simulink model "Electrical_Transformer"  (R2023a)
settings: Solver=VariableStepAuto  StartTime=0.0  StopTime=10.0  RelTol=1e-3
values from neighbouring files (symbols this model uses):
  R = 1    [Electrical_Transformer_EQN.m]    (also in Electrical_Transformer_SLX_m.m; Mechanical_Transmission_EQN.m; Mechanical_Transmission_SLX_m.m; Mechanical_system_EQN.m)
undefined symbols (not defined in the file or in its folder): eTe
libraries: fl_lib x9

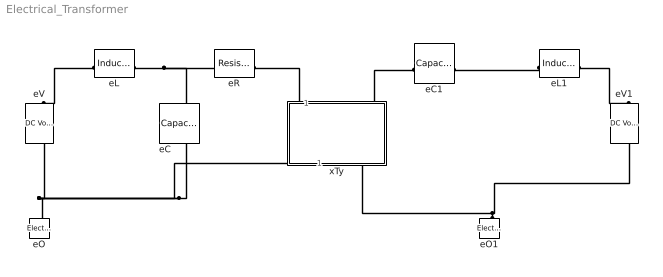
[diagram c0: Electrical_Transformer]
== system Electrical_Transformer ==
  eC : fl_lib/Electrical/Electrical Elements/Capacitor  c=1e-6 F  r=1e-6 Ohm  g=0 1/Ohm  i_specify=off  i_priority=None  i=0 A  i_nominal_specify=off  i_nominal_unit=A  i_nominal_value=1  v_specify=off  v_priority=None  v=0 V  v_nominal_specify=off  v_nominal_unit=V  v_nominal_value=1  vc_specify=off  vc_priority=High  vc=0 V  vc_nominal_specify=off  vc_nominal_unit=V  vc_nominal_value=1
  eC1 : fl_lib/Electrical/Electrical Elements/Capacitor  c=1e-6 F  r=1e-6 Ohm  g=0 1/Ohm  i_specify=off  i_priority=None  i=0 A  i_nominal_specify=off  i_nominal_unit=A  i_nominal_value=1  v_specify=off  v_priority=None  v=0 V  v_nominal_specify=off  v_nominal_unit=V  v_nominal_value=1  vc_specify=off  vc_priority=High  vc=0 V  vc_nominal_specify=off  vc_nominal_unit=V  vc_nominal_value=1
  eL : fl_lib/Electrical/Electrical Elements/Inductor  l=1e-6 H  r=0 Ohm  g=1e-9 1/Ohm  i_specify=off  i_priority=None  i=0 A  i_nominal_specify=off  i_nominal_unit=A  i_nominal_value=1  v_specify=off  v_priority=None  v=0 V  v_nominal_specify=off  v_nominal_unit=V  v_nominal_value=1  i_L_specify=off  i_L_priority=High  i_L=0 A  i_L_nominal_specify=off  i_L_nominal_unit=A  i_L_nominal_value=1
  eL1 : fl_lib/Electrical/Electrical Elements/Inductor  l=1e-6 H  r=0 Ohm  g=1e-9 1/Ohm  i_specify=off  i_priority=None  i=0 A  i_nominal_specify=off  i_nominal_unit=A  i_nominal_value=1  v_specify=off  v_priority=None  v=0 V  v_nominal_specify=off  v_nominal_unit=V  v_nominal_value=1  i_L_specify=off  i_L_priority=High  i_L=0 A  i_L_nominal_specify=off  i_L_nominal_unit=A  i_L_nominal_value=1
  eO : fl_lib/Electrical/Electrical Elements/Electrical Reference
  eO1 : fl_lib/Electrical/Electrical Elements/Electrical Reference
  eR : fl_lib/Electrical/Electrical Elements/Resistor  R=1 Ohm  i_specify=off  i_priority=None  i=0 A  i_nominal_specify=off  i_nominal_unit=A  i_nominal_value=1  v_specify=off  v_priority=None  v=0 V  v_nominal_specify=off  v_nominal_unit=V  v_nominal_value=1
  eV : fl_lib/Electrical/Electrical Sources/DC Voltage Source  v0=1 V
  eV1 : fl_lib/Electrical/Electrical Sources/DC Voltage Source  v0=1 V
  xTy : Subsystem  mask{Transformer_type=eTe, T_type=E2=K*E1, xTy=R}
      mask prompts: Transformer_type "Type of Transformer"; T_type "Type of relation"; xTy "Name of parameter K"
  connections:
  xTy/RConn1 -- eC/RConn1 -- eV/RConn1 -- eO/LConn1
  eL/LConn1 -- eV/LConn1
  eL/RConn1 -- eR/LConn1 -- eC/LConn1
  eL1/LConn1 -- eC1/RConn1
  eO1/LConn1 -- xTy/RConn2 -- eV1/RConn1
  eL1/RConn1 -- eV1/LConn1
  eR/RConn1 -- xTy/LConn1
  eC1/LConn1 -- xTy/LConn2

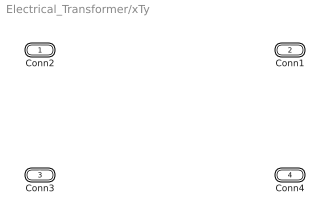
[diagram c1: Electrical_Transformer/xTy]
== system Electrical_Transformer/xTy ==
  Conn2 : PMIOPort  Side=Left
  Conn1 : PMIOPort  Port=2  Side=Left
  Conn3 : PMIOPort  Port=3  Side=Right
  Conn4 : PMIOPort  Port=4  Side=Right
